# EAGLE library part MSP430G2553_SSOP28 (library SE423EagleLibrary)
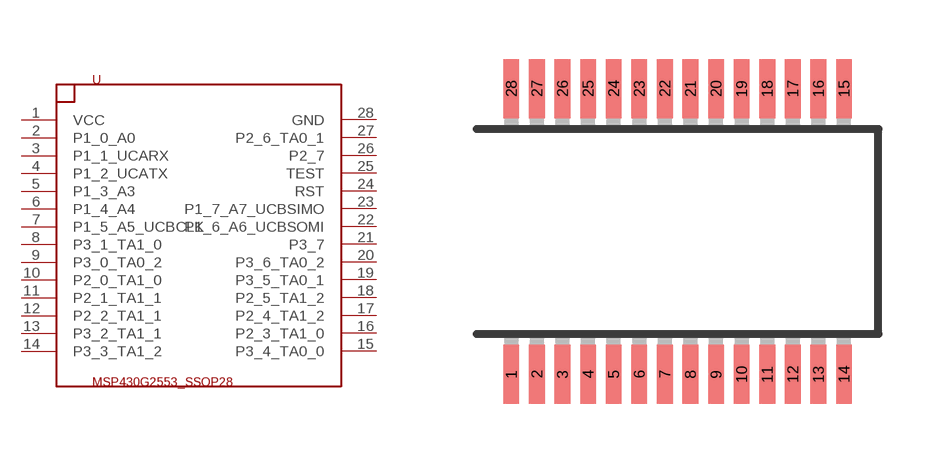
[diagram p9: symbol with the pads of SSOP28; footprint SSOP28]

Designator prefix U

## MSP430G2553_SSOP28  [SSOP28]
1  VCC
2  P1_0_A0
3  P1_1_UCARX
4  P1_2_UCATX
5  P1_3_A3
6  P1_4_A4
7  P1_5_A5_UCBCLK
8  P3_1_TA1_0
9  P3_0_TA0_2
10  P2_0_TA1_0
11  P2_1_TA1_1
12  P2_2_TA1_1
13  P3_2_TA1_1
14  P3_3_TA1_2
15  P3_4_TA0_0
16  P2_3_TA1_0
17  P2_4_TA1_2
18  P2_5_TA1_2
19  P3_5_TA0_1
20  P3_6_TA0_2
21  P3_7
22  P1_6_A6_UCBSOMI
23  P1_7_A7_UCBSIMO
24  RST
25  TEST
26  P2_7
27  P2_6_TA0_1
28  GND

## Footprint SSOP28 (pad centres in mm)
Shrink Small Outline Package package type SS
smd 0.4 x 1.5: 1 -4.225,-3.625; 2 -3.575,-3.625; 3 -2.925,-3.625; 4 -2.275,-3.625; 5 -1.625,-3.625; 6 -0.975,-3.625; 7 -0.325,-3.625; 8 0.325,-3.625; 9 0.975,-3.625; 10 1.625,-3.625; 11 2.275,-3.625; 12 2.925,-3.625; 13 3.575,-3.625; 14 4.225,-3.625; 15 4.225,3.625; 16 3.575,3.625; 17 2.925,3.625; 18 2.275,3.625; 19 1.625,3.625; 20 0.975,3.625; 21 0.325,3.625; 22 -0.325,3.625; 23 -0.975,3.625; 24 -1.625,3.625; 25 -2.275,3.625; 26 -2.925,3.625; 27 -3.575,3.625; 28 -4.225,3.625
